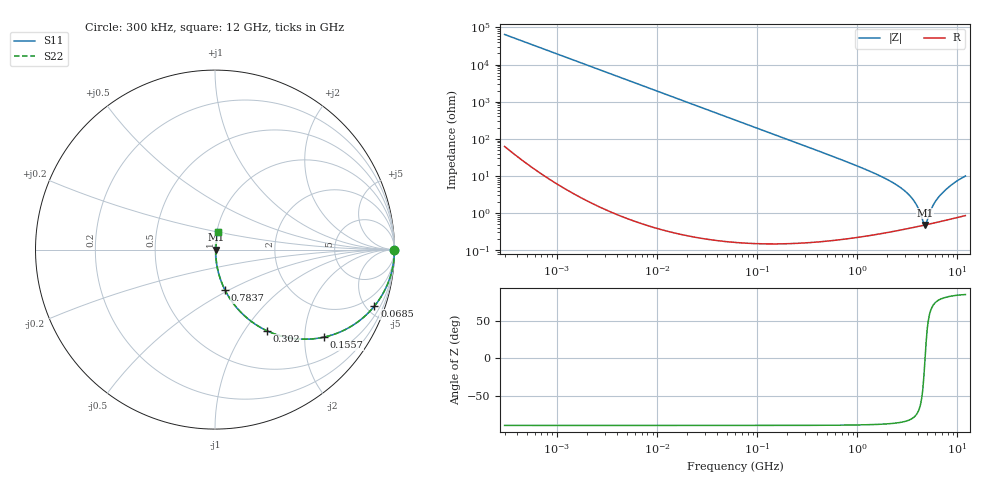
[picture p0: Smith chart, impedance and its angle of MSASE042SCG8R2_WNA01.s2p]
! MSASE042SCG8R2_WNA01  S-PARAMETER MODEL  ( General Type )
! Model Generated by TAIYO YUDEN Corporation (http://www.ty-top.com)
! Version 1.0
! TAIYO YUDEN Control No. 130801
! Copyright(c) 2013 TAIYO YUDEN CO.,LTD. All Rights Reserved.
! Product Description (link to TY-COMPAS)
! https://ds.yuden.co.jp/TYCOMPAS/or/detail?pn=MSASE042SCG8R2BWNA01&u=M
! Products Name : Multilayer Ceramic Capacitors
! Characteristics :
!  Capacitance : 8.2 pF , Rated Voltage : 16V , TCC : CG / C0G
!  Case Size : 0.4 x 0.2 / 0.016 x 0.008 [mm/inch] , Thickness : 0.2 / 0.008 [mm/inch]
!  (Conditions: Temperature = 25 degC , DC Bias Current/Voltage = 0A / 0V)
! External Node Assignments :
!  1  o---| |---o  2
! GND o---------o GND
! Frequency Range : 0.3MHz  -  12000MHz  [ 401 STEP ]
# MHz S RI R 50
! Freq[MHz].  S11 Real  S11 Imag  S21 Real  S21 Imag  S12 Real  S12 Imag  S22 Real  S22 Imag
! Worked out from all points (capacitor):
!   401 points, 300 kHz to 12 GHz, reference 50 ohm
!   read as one part in series: C = 8.22 pF near 316.3 kHz
!   lowest |Z| = 478 mohm at 4.748 GHz (marker M1)
!   series resonance near 4.745 GHz, so ESL is about 140 pH
!   S11 on the Smith chart (normalised r, x): 300 kHz: open; 68.5 MHz: 1.00, -5.65; 155.7 MHz: 1.00, -2.48; 302 MHz: 1.00, -1.28; 783.7 MHz: 1.00, -0.48; 12 GHz: 1.02, +0.20
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0.3  1 -0.00155  3.89e-06 0.00155  3.89e-06 0.00155  1 -0.00155
1.769972  0.9999 -0.00914  8.56e-05 0.00914  8.56e-05 0.00914  0.9999 -0.00914
10.44266  0.9971 -0.0538  0.00291 0.0538  0.00291 0.0538  0.9971 -0.0538
27.10171  0.9808 -0.1372  0.0192 0.1372  0.0192 0.1372  0.9808 -0.1372
60  0.9123 -0.2826  0.0877 0.2826  0.0877 0.2826  0.9123 -0.2826
68.49786  0.8886 -0.3143  0.1114 0.3143  0.1114 0.3143  0.8886 -0.3143
101.9188  0.7828 -0.412  0.2172 0.412  0.2172 0.412  0.7828 -0.412
155.7172  0.6067 -0.4879  0.3933 0.4879  0.3933 0.4879  0.6067 -0.4879
301.9711  0.2902 -0.4526  0.7098 0.4526  0.7098 0.4526  0.2902 -0.4526
353.9943  0.2291 -0.4187  0.7709 0.4187  0.7709 0.4187  0.2291 -0.4187
783.7017  0.0563 -0.2264  0.9437 0.2264  0.9437 0.2264  0.0563 -0.2264
2088.533  0.00855 -0.0739  0.9914 0.0739  0.9914 0.0739  0.00855 -0.0739
2795.104  0.00556 -0.0448  0.9944 0.0448  0.9944 0.0448  0.00556 -0.0448
3454.93  0.00465 -0.0261  0.9953 0.0261  0.9953 0.0261  0.00465 -0.0261
3944.255  0.0045 -0.015  0.9955 0.015  0.9955 0.015  0.0045 -0.015
4502.883  0.00463 -0.00417  0.9954 0.00417  0.9954 0.00417  0.00463 -0.00417
4747.894  0.00476 4.32e-05  0.9952 -4.32e-05  0.9952 -4.32e-05  0.00476 4.32e-05
5006.236  0.00493 0.00425  0.9951 -0.00425  0.9951 -0.00425  0.00493 0.00425
5715.274  0.00554 0.0152  0.9945 -0.0152  0.9945 -0.0152  0.00554 0.0152
6699.894  0.0067 0.0291  0.9933 -0.0291  0.9933 -0.0291  0.0067 0.0291
8966.534  0.0106 0.0595  0.9894 -0.0595  0.9894 -0.0595  0.0106 0.0595
12000  0.0181 0.0969  0.9819 -0.0969  0.9819 -0.0969  0.0181 0.0969
